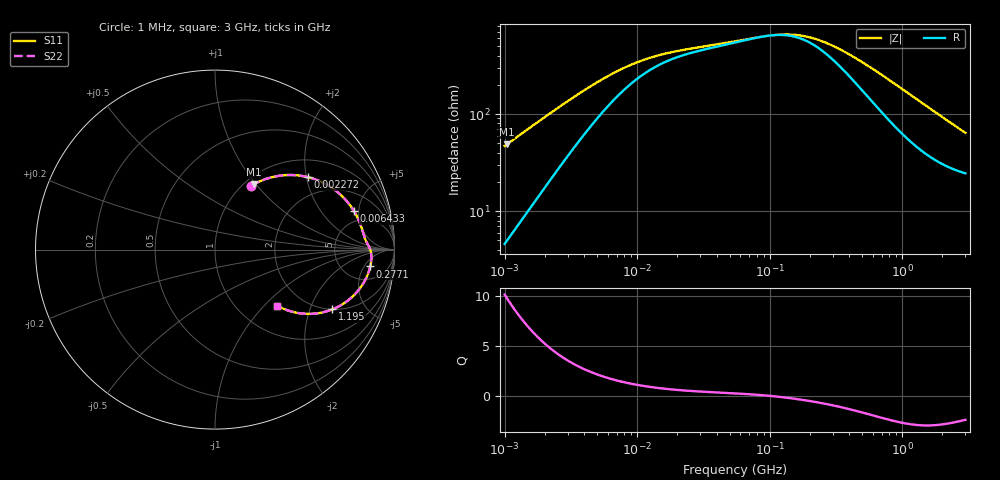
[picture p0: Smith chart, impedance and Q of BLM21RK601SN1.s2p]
! BLM21RK601SN1
# Hz S RI R 50
!Freq.(Hz) S11(Real) S11(Imag) S21(Real) S21(Imag) S12(Real) S12(Imag) S22(Real) S22(Imag)
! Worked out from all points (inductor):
!   401 points, 1 MHz to 3 GHz, reference 50 ohm
!   read as one part in series: L = 7.39 uH near 1.041 MHz
!   highest Q = 9.79 at 1.041 MHz (marker M1), where L = 7.43 uH
!   self-resonance near 97.83 MHz
!   S11 on the Smith chart (normalised r, x): 1 MHz: 1.09, +0.93; 2.272 MHz: 1.44, +2.05; 6.433 MHz: 3.66, +4.43; 277.1 MHz: 9, -7; 1.195 GHz: 2.00, -2.89; 3 GHz: 1.49, -1.18
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1000000  0.203 0.356  0.797 -0.356  0.797 -0.356  0.203 0.356
1040844  0.2155 0.3632  0.7845 -0.3632  0.7845 -0.3632  0.2155 0.3632
1553251  0.3634 0.4122  0.6366 -0.4122  0.6366 -0.4122  0.3634 0.4122
2271982  0.5189 0.4033  0.4811 -0.4033  0.4811 -0.4033  0.5189 0.4033
2947212  0.6124 0.3674  0.3876 -0.3674  0.3876 -0.3674  0.6124 0.3674
3823119  0.6859 0.3178  0.3141 -0.3178  0.3141 -0.3178  0.6859 0.3178
4861065  0.7354 0.2686  0.2646 -0.2686  0.2646 -0.2686  0.7354 0.2686
6433254  0.7743 0.2145  0.2257 -0.2145  0.2257 -0.2145  0.7743 0.2145
9794439  0.8071 0.1486  0.1929 -0.1486  0.1929 -0.1486  0.8071 0.1486
1.461624e7  0.8225 0.1038  0.1775 -0.1038  0.1775 -0.1038  0.8225 0.1038
2.225279e7  0.832 0.0718  0.168 -0.0718  0.168 -0.0718  0.832 0.0718
5.477226e7  0.8509 0.0299  0.1491 -0.0299  0.1491 -0.0299  0.8509 0.0299
1.219755e8  0.8687 -0.015  0.1313 0.015  0.1313 0.015  0.8687 -0.015
1.614254e8  0.8711 -0.0375  0.1289 0.0375  0.1289 0.0375  0.8711 -0.0375
2.094008e8  0.8703 -0.0623  0.1297 0.0623  0.1297 0.0623  0.8703 -0.0623
2.771263e8  0.865 -0.094  0.135 0.094  0.135 0.094  0.865 -0.094
4.951867e8  0.831 -0.1799  0.169 0.1799  0.169 0.1799  0.831 -0.1799
8.005644e8  0.7593 -0.2681  0.2407 0.2681  0.2407 0.2681  0.7593 -0.2681
1.194682e9  0.654 -0.333  0.346 0.333  0.346 0.333  0.654 -0.333
1.488926e9  0.5801 -0.3535  0.4199 0.3535  0.4199 0.3535  0.5801 -0.3535
1.855641e9  0.501 -0.3576  0.499 0.3576  0.499 0.3576  0.501 -0.3576
3e9  0.3451 -0.3115  0.6549 0.3115  0.6549 0.3115  0.3451 -0.3115
